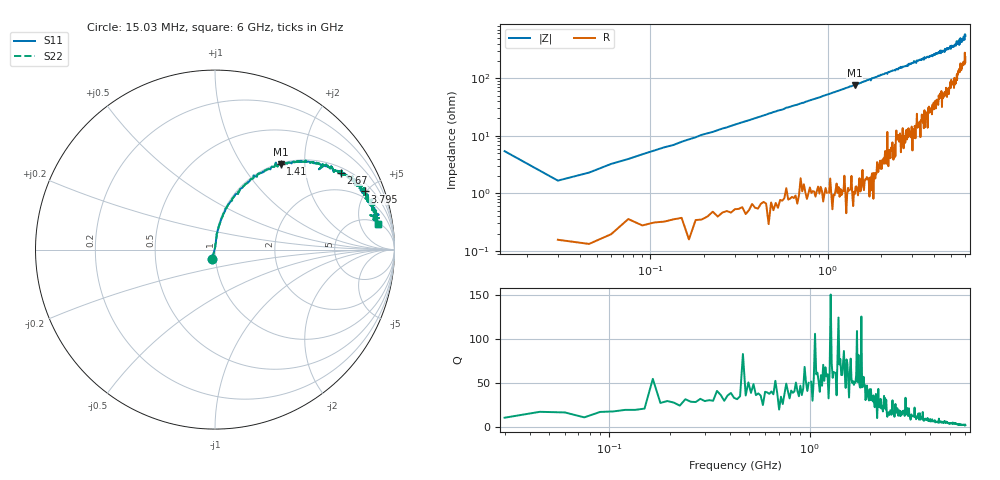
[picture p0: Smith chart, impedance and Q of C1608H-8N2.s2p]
!	Network	Analyzer	HP8753E.07.74:	Oct	30	2002	Serial	No.	JP38451487
!	Hewlett-Packard
!	7	Sep	2009	10:15:06
!	Frequency	S11	S21	S12	S22
#	HZ	S	RI	R	50
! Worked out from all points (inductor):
!   400 points, 15.03 MHz to 6 GHz, reference 50 ohm
!   read as one part in series: L = 8.34 nH near 45.03 MHz
!   highest Q = 72.7 at 1.425 GHz (marker M1), where L = 8.44 nH
!   S11 on the Smith chart (normalised r, x): 15.03 MHz: 0.96, -0.10; 1.41 GHz: 1.02, +1.52; 2.67 GHz: 1.18, +3.15; 3.795 GHz: 1.51, +4.88; 6 GHz: 6, +10
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1.502992e7  -0.0153 -0.0521  1.02 0.0521  1.02 0.0521  -0.0153 -0.0521
3.002985e7  0.00166 0.0165  0.998 -0.0165  0.998 -0.0165  0.00166 0.0165
6.00297e7  0.00297 0.0322  0.997 -0.0322  0.997 -0.0322  0.00297 0.0322
1.200294e8  0.00728 0.0624  0.993 -0.0624  0.993 -0.0624  0.00728 0.0624
2.850286e8  0.0258 0.144  0.974 -0.144  0.974 -0.144  0.0258 0.144
5.850271e8  0.0956 0.275  0.904 -0.275  0.904 -0.275  0.0956 0.275
1.020025e9  0.225 0.408  0.775 -0.408  0.775 -0.408  0.225 0.408
1.410023e9  0.367 0.475  0.633 -0.475  0.633 -0.475  0.367 0.475
1.425023e9  0.365 0.475  0.635 -0.475  0.635 -0.475  0.365 0.475
2.01002e9  0.563 0.48  0.437 -0.48  0.437 -0.48  0.563 0.48
2.670017e9  0.703 0.429  0.297 -0.429  0.297 -0.429  0.703 0.429
3.015015e9  0.767 0.408  0.233 -0.408  0.233 -0.408  0.767 0.408
3.795011e9  0.833 0.324  0.167 -0.324  0.167 -0.324  0.833 0.324
4.00501e9  0.849 0.307  0.151 -0.307  0.151 -0.307  0.849 0.307
5.010005e9  0.879 0.229  0.121 -0.229  0.121 -0.229  0.879 0.229
5.295004e9  0.887 0.223  0.113 -0.223  0.113 -0.223  0.887 0.223
5.355003e9  0.913 0.194  0.0873 -0.194  0.0873 -0.194  0.913 0.194
5.535002e9  0.865 0.192  0.135 -0.192  0.135 -0.192  0.865 0.192
5.595002e9  0.876 0.189  0.124 -0.189  0.124 -0.189  0.876 0.189
5.625002e9  0.904 0.158  0.0959 -0.158  0.0959 -0.158  0.904 0.158
5.715001e9  0.888 0.18  0.112 -0.18  0.112 -0.18  0.888 0.18
6e9  0.906 0.14  0.0943 -0.14  0.0943 -0.14  0.906 0.14
